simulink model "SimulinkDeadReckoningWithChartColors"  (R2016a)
settings: Solver=FixedStepAuto  StartTime=0.0  StopTime=inf  RelTol=1e-3
libraries: miniQ x2

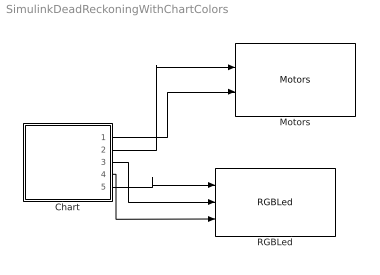
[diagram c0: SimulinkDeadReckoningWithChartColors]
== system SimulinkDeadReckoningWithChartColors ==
  Chart : Stateflow chart  TreatAsAtomicUnit=on
  Motors : miniQ/Motors  flipLeft=off  flipRight=off
  RGBLed : miniQ/RGBLed
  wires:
  Chart/2(l) -> Motors/1
  Chart/1(r) -> Motors/2
  Chart/5(red) -> RGBLed/1
  Chart/3(g) -> RGBLed/2
  Chart/4(b) -> RGBLed/3

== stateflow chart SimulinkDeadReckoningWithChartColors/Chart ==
  state Experiment with changing the "after(int,sec) function and also the values for r and l to get the dead reckoing patter you desire [group]
  state Forward
    entry: r=255
    l=255
    red=255;
    g=0;
    b=0;
  state Right
    entry: r=-255
    l=255
    red=255;
    g=0;
    b=0;
  state Forward2
    entry: r=255
    l=255
    red=255;
    g=0;
    b=0;
  state Stop
    entry: r=0
    l=0
    red=255;
    g=0;
    b=0;
  state Left
    entry: r=255
    l=-255
    red=255;
    g=255;
    b=0;
  state Forward1
    entry: r=255
    l=255
    red=0;
    g=255;
    b=0;
  (default) -> Forward
  Forward2 -> Stop : after(2,sec)
  Right -> Forward2 : after(1,sec)
  Forward1 -> Right : after(1,sec)
  Forward -> Left : after(2,sec)
  Left -> Forward1 : after(1,sec)
  data: r output; l output; g output; b output; red output
